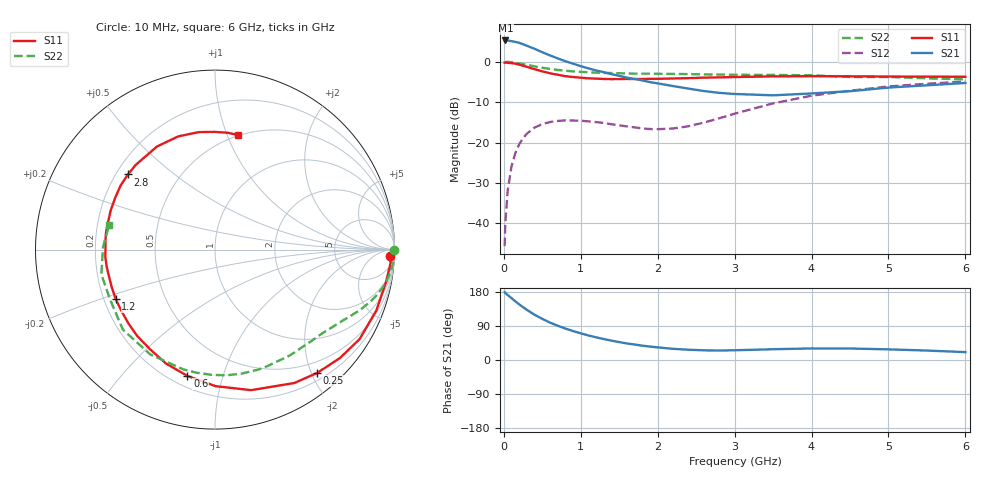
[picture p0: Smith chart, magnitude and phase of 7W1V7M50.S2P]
! Infineon Technologies  Discrete & RF Semiconductors
! BFS17W
! Si NPN RF Bipolar Junction Transistor in SOT323
! VCE = 1.75 V  IC = 0.5 mA
! Common Emitter S-Parameters:  August  1999
# GHz  S  MA  R  50
!  f  S11  S21  S12  S22
! GHz  MAG  ANG  MAG  ANG  MAG  ANG  MAG  ANG
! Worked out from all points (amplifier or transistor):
!   36 points, 10 MHz to 6 GHz, reference 50 ohm
!   highest |S21| = 5.3 dB at 20 MHz (marker M1)
!   |S21| within 3 dB of that: start of sweep to 510.3 MHz
!   unconditionally stable (mu >= 1): 1.15 GHz to end of sweep
!   at 250 MHz: K = 0.24, MSG = 11.6 dB, |S12| = -18.9 dB
!   at 1.4 GHz: K = 1.20, MAG = 3.5 dB, |S12| = -15.5 dB
!   at 6 GHz: K = 1.11, MAG = -2.2 dB, |S12| = -4.9 dB
!   S11 on the Smith chart (normalised r, x): 10 MHz: 27, -39; 250 MHz: 0.31, -2.09; 600 MHz: 0.26, -0.77; 1.2 GHz: 0.25, -0.22; 2.8 GHz: 0.25, +0.35; 6 GHz: 0.50, +1.10
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0.01  0.9765 -2.0  1.83 179.1  0.0052 86.1  0.9999 -0.2
0.02  0.981 -4.5  1.836 176.7  0.0103 91.7  0.9855 -1.3
0.05  0.9702 -10.6  1.834 171.4  0.0254 84.0  0.9952 -3.5
0.1  0.9607 -20.7  1.8 163.3  0.0508 77.6  0.9884 -6.9
0.2  0.9216 -41.0  1.715 146.8  0.0953 65.2  0.9557 -13.0
0.25  0.8923 -50.4  1.647 139.3  0.1131 59.1  0.9358 -15.8
0.3  0.8645 -59.3  1.578 132.3  0.1289 54.7  0.9166 -18.1
0.4  0.8085 -75.6  1.446 119.3  0.1531 45.9  0.8766 -22.5
0.5  0.7607 -89.8  1.312 108.5  0.169 39.0  0.8424 -25.9
0.6  0.7204 -102.3  1.198 98.7  0.1793 33.4  0.8147 -29.0
0.8  0.6628 -123.1  1.017 83.0  0.1879 25.2  0.7745 -34.9
1.1  0.6229 -147.2  0.829 64.7  0.1827 18.4  0.7409 -43.3
1.2  0.6182 -153.4  0.78 59.8  0.1787 17.0  0.7326 -46.3
1.6  0.6126 -176.0  0.636 43.6  0.1582 18.3  0.7161 -58.5
2.2  0.6207 159.6  0.5 29.5  0.1491 37.3  0.7067 -78.1
2.8  0.6407 139.2  0.412 25.1  0.1995 54.4  0.6935 -98.5
3.5  0.659 119.4  0.384 28.4  0.3053 56.2  0.6867 -121.6
4  0.6632 108.0  0.405 30.5  0.3799 50.8  0.6799 -139.0
4.5  0.6608 97.9  0.432 30.3  0.4373 44.3  0.6473 -154.6
5  0.6559 90.3  0.479 28.1  0.4944 37.9  0.6482 -167.7
5.5  0.6549 83.7  0.511 24.9  0.5342 31.6  0.624 178.8
6  0.651 78.4  0.546 20.8  0.5703 25.8  0.6059 167.0
